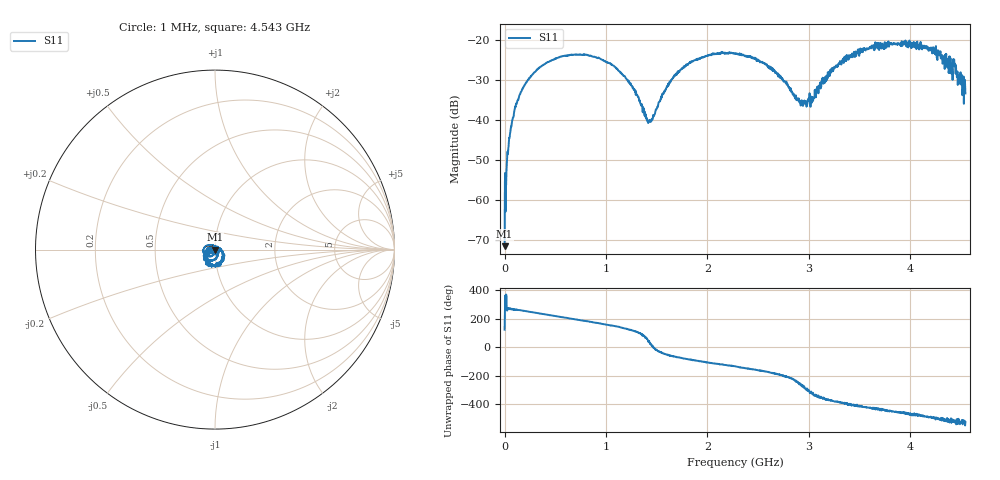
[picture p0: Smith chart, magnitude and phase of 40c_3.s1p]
# HZ S RI R 50
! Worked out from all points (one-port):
!   1515 points, 1 MHz to 4.543 GHz, reference 50 ohm
!   lowest |S11| = -71.5 dB at 1 MHz (marker M1), VSWR 1.00, Z = 50 + j0.0224 ohm
!   |S11| at or under -10 dB: start of sweep to end of sweep
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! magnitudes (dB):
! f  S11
! 1 MHz  -71.5
! 25 MHz  -49.7
! 43 MHz  -45.7
! 85 MHz  -39.3
! 127 MHz  -35.2
! 193 MHz  -31.5
! 310 MHz  -27.7
! 571 MHz  -24.0
! 910 MHz  -24.4
! 1.138 GHz  -27.9
! 1.27 GHz  -32.1
! 1.429 GHz  -40.0
! 1.609 GHz  -31.6
! 1.705 GHz  -28.3
! 2.002 GHz  -24.0
! 2.272 GHz  -23.4
! 2.566 GHz  -25.8
! 2.842 GHz  -33.6
! 2.926 GHz  -35.1
! 3.034 GHz  -34.3
! 3.208 GHz  -27.5
! 3.409 GHz  -23.7
! 3.664 GHz  -21.2
! 3.976 GHz  -21.5
! 4.291 GHz  -23.1
! 4.396 GHz  -24.5
! 4.441 GHz  -25.9
! 4.543 GHz  -33.3
